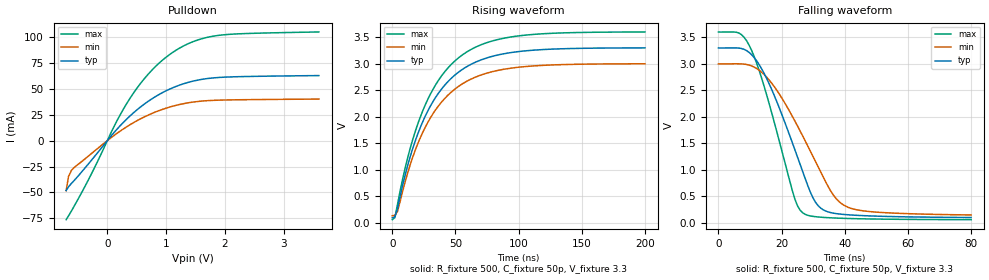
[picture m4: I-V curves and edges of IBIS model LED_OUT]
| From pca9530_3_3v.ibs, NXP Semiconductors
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[Model]   LED_OUT
Model_type Open_drain
Vref=3.3
Vmeas=1.65
Rref=500
Cref=50p
C_comp   5p   4.8p   5.2p
[Temperature Range] 27   85   -40
[Voltage Range]   3.3   3   3.6
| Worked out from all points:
|   slope of the pulldown table from 0 to 0.495 V, typ, clamps not added: 16.9 ohm
|   falling waveform, R_fixture 500, C_fixture 50p, V_fixture 3.3: 20-80 % time 12.3ns typ, 15.2ns min, 9.88ns max; typ from 3.3 V to 0.104 V
|   rising waveform, R_fixture 500, C_fixture 50p, V_fixture 3.3: 20-80 % time 35.4ns typ, 35.5ns min, 35.3ns max; typ from 0.093 V to 3.3 V
[Pulldown]
-700mV    -48.11mA   -48.26mA   -76.24mA
-660mV    -44.53mA   -34.57mA   -72.62mA
-610mV    -41.24mA   -28.67mA   -67.81mA
-570mV    -38.82mA   -26.24mA   -63.82mA
-270mV    -18.91mA   -12.45mA   -32.05mA
130mV     8.828mA    5.64mA     15.38mA
340mV     21.34mA    13.74mA    36.68mA
690mV     37.72mA    24.5mA     63.74mA
1.04V     49.18mA    32.04mA    82.21mA
1.43V     57.02mA    36.98mA    94.82mA
1.82V     60.61mA    38.91mA    101mA
3.6V      62.78mA    40.11mA    104.8mA
[Falling Waveform]
R_fixture=500
C_fixture=50p
V_fixture=3.3
V_fixture_min=3
V_fixture_max=3.6
0s        3.3V       3V         3.6V
6.465ns   3.298V     3.001V     3.582V
10.51ns   3.174V     2.961V     3.255V
16.97ns   2.503V     2.628V     2.055V
24.24ns   1.375V     1.919V     443.7mV
26.67ns   972.4mV    1.642V     193.3mV
31.52ns   331.1mV    1.067V     114.6mV
36.36ns   186.2mV    529.9mV    95.83mV
40.4ns    158.2mV    313.9mV    86.83mV
80ns      103.5mV    152mV      62.92mV
[Rising Waveform]
R_fixture=500
C_fixture=50p
V_fixture=3.3
V_fixture_min=3
V_fixture_max=3.6
0s        93.22mV    132.3mV    58.12mV
2.02ns    109.4mV    140.1mV    96.37mV
4.04ns    253.5mV    207.8mV    336mV
14.14ns   1.244V     1.092V     1.401V
24.24ns   1.914V     1.712V     2.119V
38.38ns   2.503V     2.259V     2.75V
54.55ns   2.877V     2.606V     3.149V
72.73ns   3.093V     2.807V     3.38V
98.99ns   3.226V     2.931V     3.521V
200ns     3.299V     2.999V     3.599V
[Ramp]
R_load=500
dV/dt_r   1.924E+0/1.288E-9   1.892E+0/1.844E-9   1.948E+0/9.353E-10
dV/dt_f   1.924E+0/1.010E-8   1.892E+0/1.344E-8   1.948E+0/7.762E-9
|[End   LED_OUT
